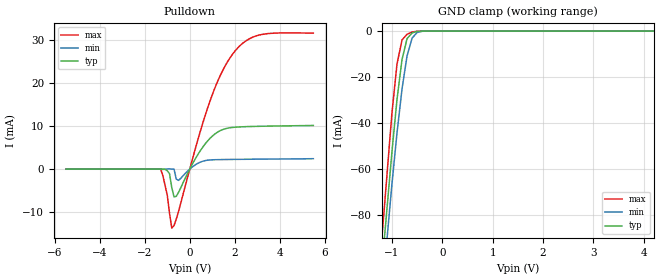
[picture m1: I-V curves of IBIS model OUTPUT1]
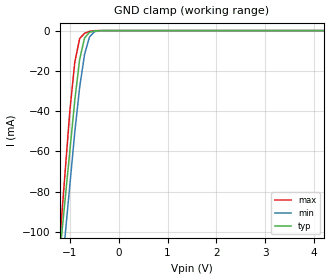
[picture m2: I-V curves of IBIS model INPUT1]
| IBIS file 4045nb.ibs
[IBIS ver]   3.2
[File name]   4045nb.ibs
[File Rev]   1.0
[Date]   Jul 19, 2012
[Source]   This file orginated at SEIKO EPSON QD Div.
[Copyright]   Copyright SEIKO EPSON Corp. 2012
|   Component 4045nb
[Component]   4045nb
[Manufacturer]   SEIKO EPSON
[Package]
| variable   typ   min   max
R_pkg   87m   NA   NA
L_pkg   10nH   NA   NA
C_pkg   206fF   NA   NA
[Pin]  signal_name   model_name   R_pin   L_pin   C_pin
|1   CE
2   VDD   POWER
|3   (GNG)
|4   TEST
5   FOUT   OUTPUT1
6   CLK   INPUT1
|7   DO
|8   DI
9   GND   GND
| Models and submodels in the file (2): OUTPUT1 (Open_drain), INPUT1 (Input)
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|10   /INT
|11   NC
|12   NC
|13   NC
|14   NC
|15   NC
|16   NC
|17   NC
|18   NC
|19   NC
|20   NC
|21   NC
|22   NC
|   Model OUTPUT
[Model]   OUTPUT1
Model_type   Open_drain
Polarity   Non-Inverting
Vmeas =   1.50V
C_comp   1.69pF   1.32pF   1.96pF
[Temperature Range]   25.00   85.00   -40.000
[Voltage Range]   3.0V   1.7V   5.5V
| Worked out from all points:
|   slope of the pulldown table from 0 to 0.45 V, typ, clamps not added: 110 ohm
|   GND clamp passes 1 mA (typ) near -0.61 V on its own axis
[Pulldown]
| voltage   I(typ)   I(min)   I(max)
-5.5V     0A         0A         0A
-1.3V     0A         0A         0A
-1V       -388uA     25uA       -6.092mA
-900mV    -1.083mA   53uA       -10.3mA
-800mV    -4.316mA   -17uA      -13.73mA
-700mV    -6.466mA   -23uA      -13.11mA
-600mV    -6.33mA    -2.33mA    -11.61mA
300mV     2.853mA    1.155mA    5.703mA
900mV     7.133mA    2.119mA    15.8mA
1.9V      9.676mA    2.242mA    26.66mA
3.1V      9.938mA    2.303mA    31.15mA
5.5V      10.13mA    2.41mA     31.58mA
[GND_clamp]
| voltage   I(typ)   I(min)   I(max)
-5.5V     -1.182A    -1.162A    -1.261A
-1.2V     -102.7mA   -115.2mA   -90.08mA
-1.1V     -77.56mA   -90.84mA   -62.86mA
-1V       -52.45mA   -66.5mA    -35.63mA
-900mV    -29.83mA   -44.41mA   -14.39mA
-800mV    -12.38mA   -25.18mA   -3.855mA
-700mV    -3.281mA   -10.8mA    -1.386mA
-600mV    -820uA     -3.055mA   -435uA
-500mV    -190uA     -606uA     -49uA
-300mV    0A         -7uA       0A
5.5V      0A         0A         0A
[Ramp]
| variable   typ   min   max
dV/dt_r 1.968/4.56n   0.874/16.96n   3.888/1.422n
dV/dt_f 1.968/4.56n   0.874/16.96n   3.888/1.422n
R_load = 500.00
| End [Model] OUTPUT
|   Model INPUT1
[Model]   INPUT1
Model_type   Input
Polarity   Non-Inverting
Vinl = 0.60V
Vinh = 2.40V
C_comp   0.80pF   0.60pF   1.00pF
[Temperature Range]   25.00   85.00   -40.00
[Voltage Range]   3.0V   1.7V   5.5V
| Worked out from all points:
|   GND clamp passes 1 mA (typ) near -0.60 V on its own axis
[GND_clamp]
| voltage   I(typ)   I(min)   I(max)
-5.5V     -1.179A    -1.245A    -1.443A
-1.2V     -109.2mA   -128.4mA   -102mA
-1.1V     -84.36mA   -102.4mA   -70.81mA
-1V       -59.47mA   -76.41mA   -39.62mA
-900mV    -34.59mA   -50.44mA   -15.66mA
-800mV    -14.24mA   -28.13mA   -3.931mA
-700mV    -3.678mA   -11.8mA    -1.351mA
-600mV    -868uA     -3.229mA   -419uA
-500mV    -202uA     -612uA     -46uA
-300mV    -1uA       -7uA       0A
5.5V      0A         0A         0A
